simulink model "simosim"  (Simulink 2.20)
settings: Solver=FixedStepDiscrete  StartTime=0.0  StopTime=50  FixedStep=1  RelTol=1e-3  AbsTol=1e-6

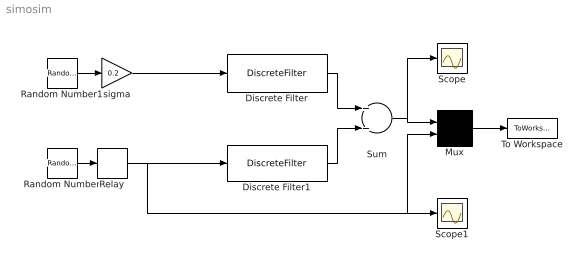
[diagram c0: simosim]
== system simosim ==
  Discrete Filter : DiscreteFilter  Numerator=[1 -1 0.2]  Denominator=[1 -1.5 0.7]  SampleTime=1
  Discrete Filter1 : DiscreteFilter  Numerator=[1 0.5]  Denominator=[1 -1.5 0.7]  SampleTime=1
  Mux : Mux  Inputs=2
  Random Number : RandomNumber  Mean=0  Variance=1  Seed=123456789  SampleTime=1
  Random Number1 : RandomNumber  Mean=0  Variance=1  Seed=123459  SampleTime=1
  Relay : Relay  OnSwitchValue=eps  OffSwitchValue=eps  OnOutputValue=-1  OffOutputValue=1
  Scope : Scope
  Scope1 : Scope
  Sum : Sum  Inputs=++
  To Workspace : ToWorkspace  VariableName=zsim  SampleTime=1
  sigma : Gain  Gain=0.2
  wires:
  Random Number/1 -> Relay/1
  Random Number1/1 -> sigma/1
  sigma/1 -> Discrete Filter/1
  Discrete Filter/1 -> Sum/1
  Discrete Filter1/1 -> Sum/2
  Sum/1 -> Scope/1, Mux/1
  Relay/1 -> Discrete Filter1/1, Mux/2, Scope1/1
  Mux/1 -> To Workspace/1
